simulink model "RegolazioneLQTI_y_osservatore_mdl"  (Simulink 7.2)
settings: Solver=ode45  StartTime=0.0  StopTime=10.0  RelTol=1e-3
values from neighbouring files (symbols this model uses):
  A = [0 1; -2 1]    [RegolazioneOttimaTempoInfinita_Integrale.m]    (also in RegolazioneOttimaTempoInfinita_TempoDiscreto.m; RegolazioneOttimaTempoInfinita_uscita.m; RegolazioneOttimaTempoInfinita_uscita_osservatore.m; RegolazioneOttimaTempoInfinita.m)
  A1 = A    [RegolazioneOttimaTempoInfinita_uscita_osservatore.m]
  B = [0; 1]    [RegolazioneOttimaTempoInfinita_Integrale.m]    (also in RegolazioneOttimaTempoInfinita_TempoDiscreto.m; RegolazioneOttimaTempoInfinita_uscita.m; RegolazioneOttimaTempoInfinita_uscita_osservatore.m; RegolazioneOttimaTempoInfinita.m)
  B1 = B    [RegolazioneOttimaTempoInfinita_uscita_osservatore.m]
  C = [1 0]    [RegolazioneOttimaTempoInfinita_Integrale.m]    (also in RegolazioneOttimaTempoInfinita_TempoDiscreto.m; RegolazioneOttimaTempoInfinita_uscita.m = [0 1]; RegolazioneOttimaTempoInfinita_uscita_osservatore.m = [0 1]; RegolazioneOttimaTempoInfinita.m)
  C1 = C    [RegolazioneOttimaTempoInfinita_uscita_osservatore.m]
  L = - acker(A1',C1',[-10 -10])'    [RegolazioneOttimaTempoInfinita_uscita_osservatore.m]
  X0 = [2;-3]    [RegolazioneOttimaTempoInfinita_Integrale.m]    (also in RegolazioneOttimaTempoInfinita_TempoDiscreto.m; RegolazioneOttimaTempoInfinita_uscita.m; RegolazioneOttimaTempoInfinita_uscita_osservatore.m; RegolazioneOttimaTempoInfinita.m)
undefined symbols (not defined in the file or in its folder): K

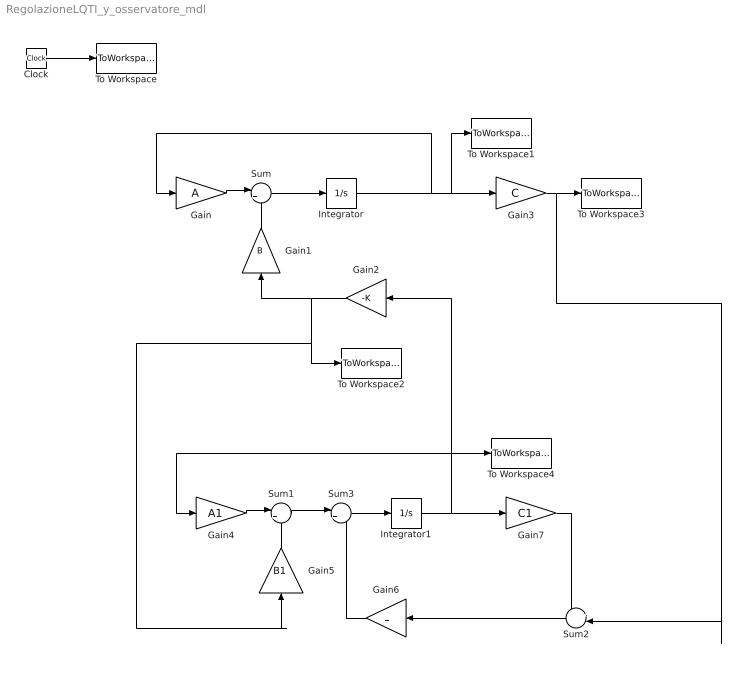
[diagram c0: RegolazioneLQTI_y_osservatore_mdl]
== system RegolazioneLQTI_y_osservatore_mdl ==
  Clock : Clock
  Gain : Gain  Gain=A  Multiplication=Matrix(K*u)  ParameterDataType=sfix(16)  ParameterScaling=2^0  OutDataType=sfix(16)  OutScaling=2^0
  Gain1 : Gain  Orientation=up  Gain=B  Multiplication=Matrix(K*u)  ParameterDataType=sfix(16)  ParameterScaling=2^0  OutDataType=sfix(16)  OutScaling=2^0
  Gain2 : Gain  Orientation=left  Gain=-K  Multiplication=Matrix(K*u)  ParameterDataType=sfix(16)  ParameterScaling=2^0  OutDataType=sfix(16)  OutScaling=2^0
  Gain3 : Gain  Gain=C  Multiplication=Matrix(K*u)  ParameterDataType=sfix(16)  ParameterScaling=2^0  OutDataType=sfix(16)  OutScaling=2^0
  Gain4 : Gain  Gain=A1  Multiplication=Matrix(K*u)  ParameterDataType=sfix(16)  ParameterScaling=2^0  OutDataType=sfix(16)  OutScaling=2^0
  Gain5 : Gain  Orientation=up  Gain=B1  Multiplication=Matrix(K*u)  ParameterDataType=sfix(16)  ParameterScaling=2^0  OutDataType=sfix(16)  OutScaling=2^0
  Gain6 : Gain  Orientation=left  Gain=L  Multiplication=Matrix(K*u)  ParameterDataType=sfix(16)  ParameterScaling=2^0  OutDataType=sfix(16)  OutScaling=2^0
  Gain7 : Gain  Gain=C1  Multiplication=Matrix(K*u)  ParameterDataType=sfix(16)  ParameterScaling=2^0  OutDataType=sfix(16)  OutScaling=2^0
  Integrator : Integrator  InitialCondition=X0
  Integrator1 : Integrator  InitialCondition=[0 0]
  Sum : Sum  Inputs=|++  OutDataType=sfix(16)  OutScaling=2^0
  Sum1 : Sum  Inputs=|++  OutDataType=sfix(16)  OutScaling=2^0
  Sum2 : Sum  Orientation=left  Inputs=+-  OutDataType=sfix(16)  OutScaling=2^0
  Sum3 : Sum  Inputs=|++  OutDataType=sfix(16)  OutScaling=2^0
  To Workspace : ToWorkspace  VariableName=time  SampleTime=-1  SaveFormat=Array
  To Workspace1 : ToWorkspace  VariableName=X  SampleTime=-1  SaveFormat=Array
  To Workspace2 : ToWorkspace  VariableName=u  SampleTime=-1  SaveFormat=Array
  To Workspace3 : ToWorkspace  VariableName=y  SampleTime=-1  SaveFormat=Array
  To Workspace4 : ToWorkspace  VariableName=X1  SampleTime=-1  SaveFormat=Array
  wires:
  Gain/1 -> Sum/1
  Integrator/1 -> Gain/1, To Workspace1/1, Gain3/1
  Gain1/1 -> Sum/2
  Gain2/1 -> Gain1/1, To Workspace2/1, Gain5/1
  Sum/1 -> Integrator/1
  Clock/1 -> To Workspace/1
  Gain3/1 -> To Workspace3/1, Sum2/2
  Gain4/1 -> Sum1/1
  Integrator1/1 -> Gain7/1, Gain4/1, Gain2/1, To Workspace4/1
  Gain5/1 -> Sum1/2
  Sum2/1 -> Gain6/1
  Gain7/1 -> Sum2/1
  Gain6/1 -> Sum3/2
  Sum1/1 -> Sum3/1
  Sum3/1 -> Integrator1/1
